FUNCTION_BLOCK FB_LN_IED_LD1_CSWI1 EXTENDS FB_AcsiCommonLogicalNodeClass
VAR_INPUT
	NamPlt: FB_DO_IED_LD1_CSWI1_NamPlt := (sClass:='LPL', bLinkResult:=THIS^.AddDataToContainer(ipData:=NamPlt));
	Beh: FB_DO_IED_LD1_CSWI1_Beh := (sClass:='ENS', bLinkResult:=THIS^.AddDataToContainer(ipData:=Beh));
	Health: FB_DO_IED_LD1_CSWI1_Health := (sClass:='ENS', bLinkResult:=THIS^.AddDataToContainer(ipData:=Health));
	Mod_: FB_DO_IED_LD1_CSWI1_Mod := (sObjectName:='Mod', sClass:='ENC', bLinkResult:=THIS^.AddDataToContainer(ipData:=Mod_));
	Pos: FB_DO_IED_LD1_CSWI1_Pos := (sClass:='DPC', bLinkResult:=THIS^.AddDataToContainer(ipData:=Pos));
END_VAR
VAR
END_VAR

END_FUNCTION_BLOCK
